ORGANIZATION_BLOCK OB 1
BEGIN
	// Check pointer immediates
	L		P#10.6
	__ASSERT==	__ACCU 1,	DW#16#00000056
	L		P#P 1.1
	__ASSERT==	__ACCU 1,	DW#16#80000009
	L		P#E 2.1
	__ASSERT==	__ACCU 1,	DW#16#81000011
	L		P#A 3.1
	__ASSERT==	__ACCU 1,	DW#16#82000019
	L		P#M 4.1
	__ASSERT==	__ACCU 1,	DW#16#83000021
	L		P#L 5.1
	__ASSERT==	__ACCU 1,	DW#16#86000029


	// Test address register instructions
	L		P#885.3
	LAR1
	L		P#886.2
	LAR2
	__ASSERT==	__ACCU 1,	P#886.2
	__ASSERT==	__ACCU 2,	P#885.3
	__ASSERT==	__AR 1,		P#885.3
	__ASSERT==	__AR 2,		P#886.2
	+AR1		P#1.1
	__ASSERT==	__AR 1,		P#886.4
	+AR2		P#5.1
	__ASSERT==	__AR 2,		P#891.3
	LAR1		P#12.3
	LAR2		P#32.1
	__ASSERT==	__AR 1,		P#12.3
	__ASSERT==	__AR 2,		P#32.1
	L		111
	L		222
	TAR1
	__ASSERT==	__ACCU 1,	P#12.3
	__ASSERT==	__ACCU 2,	222
	TAR2
	__ASSERT==	__ACCU 1,	P#32.1
	__ASSERT==	__ACCU 2,	P#12.3
	TAR1		LD 0
	TAR2		LD 4
	__ASSERT==	LD 0,		P#12.3
	__ASSERT==	LD 4,		P#32.1


	// Test indirect read
	L		0
	T		MD 100
	T		MD 104
	SET
	=		M 100.0
	=		M 100.2
	LAR1		P#100.0
	LAR2		P#104.0
	U		M [AR1, P#0.0]
	__ASSERT==	__STW VKE,	1
	U		M [AR1, P#0.1]
	__ASSERT==	__STW VKE,	0
	U		M [AR1, P#0.2]
	__ASSERT==	__STW VKE,	1
	U		M [AR1, P#0.3]
	__ASSERT==	__STW VKE,	0
	U		M [AR1, P#1.0]
	__ASSERT==	__STW VKE,	0
	U		M [AR2, P#0.0]
	__ASSERT==	__STW VKE,	0
	LAR1		P#100.1
	U		M [AR1, P#0.0]
	__ASSERT==	__STW VKE,	0
	U		M [AR1, P#0.1]
	__ASSERT==	__STW VKE,	1
	L		P#100.0
	T		LD 0
	U		M [LD 0]
	__ASSERT==	__STW VKE,	1
	L		P#100.1
	T		LD 0
	U		M [LD 0]
	__ASSERT==	__STW VKE,	0
	L		P#100.0
	T		LD 0
	L		MD [LD 0]
	__ASSERT==	__ACCU 1,	DW#16#05000000
	LAR1		P#M 100.0
	U		[AR1, P#0.0]
	__ASSERT==	__STW VKE,	1
	U		[AR1, P#0.1]
	__ASSERT==	__STW VKE,	0
	U		[AR1, P#0.2]
	__ASSERT==	__STW VKE,	1
	U		[AR1, P#0.3]
	__ASSERT==	__STW VKE,	0
	LAR1		P#M 100.0
	L		B [AR1, P#0.0]
	__ASSERT==	__ACCU 1,	DW#16#00000005
	L		W [AR1, P#0.0]
	__ASSERT==	__ACCU 1,	DW#16#00000500
	L		D [AR1, P#0.0]
	__ASSERT==	__ACCU 1,	DW#16#05000000


	// Test indirect write
	L		0
	T		MD 100
	T		MD 104
	SET
	=		M 100.0
	=		M 100.2
	LAR1		P#M 100.4
	=		[AR1, P#0.0]
	=		[AR1, P#0.1]
	L		MD 100
	__ASSERT==	__ACCU 1,	DW#16#35000000
	LAR1		P#M 100.0
	L		DW#16#ABCDEF12
	T		D [AR1, P#0.0]
	L		MD 100
	__ASSERT==	__ACCU 1,	DW#16#ABCDEF12
	T		D [AR1, P#1.0]
	L		MD 100
	__ASSERT==	__ACCU 1,	DW#16#ABABCDEF
	L		P#100.0
	T		LD 0
	L		DW#16#98765432
	T		MD [LD 0]
	L		MD 100
	__ASSERT==	__ACCU 1,	DW#16#98765432
	LAR1		P#100.0
	L		DW#16#12345678
	T		MD [AR1, P#0.0]
	L		MD 100
	__ASSERT==	__ACCU 1,	DW#16#12345678


	// Indirect counter access
	L		10
	T		LW 0
	L		Z [LW 0]
	__ASSERT==	__ACCU 1,	0
	SET
	ZV		Z 10
	CLR
	ZV		Z [LW 0]
	L		Z [LW 0]
	__ASSERT==	__ACCU 1,	1


	// Indirect timer access
	L		10
	T		LW 0
	L		T [LW 0]
	__ASSERT==	__ACCU 1,	0
	SET
	L		W#16#0999
	SI		T 10
	__SLEEP		50
	L		T [LW 0]
	__ASSERT<>	__ACCU 1,	0
	CLR
	L		W#16#0999
	SI		T [LW 0]
	L		T [LW 0]
	__SLEEP		50
	L		T [LW 0]
	__ASSERT==	__ACCU 1,	__ACCU 2


	CALL FB 1, DB 1 (
		IN_VAL_0	:= 6666,
		IN_VAL_1	:= 6767,
		ZERO_PTR_VAL	:= DW#16#0,
		ONE_PTR_VAL	:= DW#16#8,
	)

	CALL FC 1 (
		IN_VAL_0	:= 5555,
		IN_VAL_1	:= 5656,
	)

	CALL FC 2


	CALL SFC 46 // STOP CPU
END_ORGANIZATION_BLOCK


FUNCTION_BLOCK FB 1
	VAR_INPUT
		IN_VAL_0	: INT;
		IN_VAL_1	: INT;
		ZERO_PTR_VAL	: DWORD;
		ONE_PTR_VAL	: DWORD;
	END_VAR
BEGIN
	L		P##IN_VAL_0
	__ASSERT==	__ACCU 1,	DW#16#85000000
	L		P##IN_VAL_1
	__ASSERT==	__ACCU 1,	DW#16#85000010


	L		DW#16#11223344
	T		MD 0
	L		DW#16#55667788
	T		MD 4
	L		MD [#ZERO_PTR_VAL]
	__ASSERT==	__ACCU 1,	DW#16#11223344
	L		MD [#ONE_PTR_VAL]
	__ASSERT==	__ACCU 1,	DW#16#22334455


	L		DW#16#AABBCCDD
	T		MD 1
	L		1
	T		MW 12
	L		2
	T		MW 14
	CALL FB 2, DB 2 (
		IN_VAL_0	:= MD [#ONE_PTR_VAL],
		DB_VAL		:= DB [MW 14],
		FC_VAL		:= FC [MW 12],
		FB_VAL		:= FB [MW 12],
	)


	// Test all memory-indirect accesses
	AUF		DB 1
	L		P#8.0
	T		LD 0
	U		E [LD 0]
	=		E [LD 0]
	U		A [LD 0]
	=		A [LD 0]
	U		L [LD 0]
	=		L [LD 0]
	U		DIX [LD 0]
	=		DIX [LD 0]
	U		DBX [LD 0]
	=		DBX [LD 0]
	L		EB [LD 0]
	T		EB [LD 0]
	L		AB [LD 0]
	T		AB [LD 0]
	L		MB [LD 0]
	T		MB [LD 0]
	L		LB [LD 0]
	T		LB [LD 0]
	L		PEB [LD 0]
	T		PAB [LD 0]
	L		DBB [LD 0]
	T		DBB [LD 0]
	L		DIB [LD 0]
	T		DIB [LD 0]
	L		EW [LD 0]
	T		EW [LD 0]
	L		AW [LD 0]
	T		AW [LD 0]
	L		MW [LD 0]
	T		MW [LD 0]
	L		LW [LD 0]
	T		LW [LD 0]
	L		PEW [LD 0]
	T		PAW [LD 0]
	L		DBW [LD 0]
	T		DBW [LD 0]
	L		DIW [LD 0]
	T		DIW [LD 0]
	L		ED [LD 0]
	T		ED [LD 0]
	L		AD [LD 0]
	T		AD [LD 0]
	L		MD [LD 0]
	T		MD [LD 0]
	L		LD [LD 0]
	T		LD [LD 0]
	L		PED [LD 0]
	T		PAD [LD 0]
	L		DBD [LD 0]
	T		DBD [LD 0]
	L		DID [LD 0]
	T		DID [LD 0]
	L		0
	T		LW 0
	L		T [LW 0]
	L		Z [LW 0]

	// Test all register-indirect accesses
	AUF		DB 1
	LAR1		P#8.0
	U		E [AR1, P#0.0]
	=		E [AR1, P#0.0]
	LAR1		P#E 8.0
	U		[AR1, P#0.0]
	=		[AR1, P#0.0]
	LAR1		P#8.0
	U		A [AR1, P#0.0]
	=		A [AR1, P#0.0]
	LAR1		P#A 8.0
	U		[AR1, P#0.0]
	=		[AR1, P#0.0]
	LAR1		P#8.0
	U		M [AR1, P#0.0]
	=		M [AR1, P#0.0]
	LAR1		P#M 8.0
	U		[AR1, P#0.0]
	=		[AR1, P#0.0]
	LAR1		P#8.0
	U		L [AR1, P#0.0]
	=		L [AR1, P#0.0]
	LAR1		P#L 8.0
	U		[AR1, P#0.0]
	=		[AR1, P#0.0]
	LAR1		P#8.0
	U		DIX [AR1, P#0.0]
	=		DIX [AR1, P#0.0]
	LAR1		P#DIX 8.0
	U		[AR1, P#0.0]
	=		[AR1, P#0.0]
	LAR1		P#8.0
	U		DBX [AR1, P#0.0]
	=		DBX [AR1, P#0.0]
	LAR1		P#DBX 8.0
	U		[AR1, P#0.0]
	=		[AR1, P#0.0]

	LAR1		P#8.0
	L		EB [AR1, P#0.0]
	T		EB [AR1, P#0.0]
	LAR1		P#E 8.0
	L		B [AR1, P#0.0]
	T		B [AR1, P#0.0]
	LAR1		P#8.0
	L		AB [AR1, P#0.0]
	T		AB [AR1, P#0.0]
	LAR1		P#A 8.0
	L		B [AR1, P#0.0]
	T		B [AR1, P#0.0]
	LAR1		P#8.0
	L		MB [AR1, P#0.0]
	T		MB [AR1, P#0.0]
	LAR1		P#M 8.0
	L		B [AR1, P#0.0]
	T		B [AR1, P#0.0]
	LAR1		P#8.0
	L		LB [AR1, P#0.0]
	T		LB [AR1, P#0.0]
	LAR1		P#L 8.0
	L		B [AR1, P#0.0]
	T		B [AR1, P#0.0]
	LAR1		P#8.0
	L		PEB [AR1, P#0.0]
	T		PAB [AR1, P#0.0]
	LAR1		P#P 8.0
	L		B [AR1, P#0.0]
	T		B [AR1, P#0.0]
	LAR1		P#8.0
	L		DBB [AR1, P#0.0]
	T		DBB [AR1, P#0.0]
	LAR1		P#DBX 8.0
	L		B [AR1, P#0.0]
	T		B [AR1, P#0.0]
	LAR1		P#8.0
	L		DIB [AR1, P#0.0]
	T		DIB [AR1, P#0.0]
	LAR1		P#DIX 8.0
	L		B [AR1, P#0.0]
	T		B [AR1, P#0.0]

	LAR1		P#8.0
	L		EW [AR1, P#0.0]
	T		EW [AR1, P#0.0]
	LAR1		P#E 8.0
	L		W [AR1, P#0.0]
	T		W [AR1, P#0.0]
	LAR1		P#8.0
	L		AW [AR1, P#0.0]
	T		AW [AR1, P#0.0]
	LAR1		P#A 8.0
	L		W [AR1, P#0.0]
	T		W [AR1, P#0.0]
	LAR1		P#8.0
	L		MW [AR1, P#0.0]
	T		MW [AR1, P#0.0]
	LAR1		P#M 8.0
	L		W [AR1, P#0.0]
	T		W [AR1, P#0.0]
	LAR1		P#8.0
	L		LW [AR1, P#0.0]
	T		LW [AR1, P#0.0]
	LAR1		P#L 8.0
	L		W [AR1, P#0.0]
	T		W [AR1, P#0.0]
	LAR1		P#8.0
	L		PEW [AR1, P#0.0]
	T		PAW [AR1, P#0.0]
	LAR1		P#P 8.0
	L		W [AR1, P#0.0]
	T		W [AR1, P#0.0]
	LAR1		P#8.0
	L		DBW [AR1, P#0.0]
	T		DBW [AR1, P#0.0]
	LAR1		P#DBX 8.0
	L		W [AR1, P#0.0]
	T		W [AR1, P#0.0]
	LAR1		P#8.0
	L		DIW [AR1, P#0.0]
	T		DIW [AR1, P#0.0]
	LAR1		P#DIX 8.0
	L		W [AR1, P#0.0]
	T		W [AR1, P#0.0]

	LAR1		P#8.0
	L		ED [AR1, P#0.0]
	T		ED [AR1, P#0.0]
	LAR1		P#E 8.0
	L		D [AR1, P#0.0]
	T		D [AR1, P#0.0]
	LAR1		P#8.0
	L		AD [AR1, P#0.0]
	T		AD [AR1, P#0.0]
	LAR1		P#A 8.0
	L		D [AR1, P#0.0]
	T		D [AR1, P#0.0]
	LAR1		P#8.0
	L		MD [AR1, P#0.0]
	T		MD [AR1, P#0.0]
	LAR1		P#M 8.0
	L		D [AR1, P#0.0]
	T		D [AR1, P#0.0]
	LAR1		P#8.0
	L		LD [AR1, P#0.0]
	T		LD [AR1, P#0.0]
	LAR1		P#L 8.0
	L		D [AR1, P#0.0]
	T		D [AR1, P#0.0]
	LAR1		P#8.0
	L		PED [AR1, P#0.0]
	T		PAD [AR1, P#0.0]
	LAR1		P#P 8.0
	L		D [AR1, P#0.0]
	T		D [AR1, P#0.0]
	LAR1		P#8.0
	L		DBD [AR1, P#0.0]
	T		DBD [AR1, P#0.0]
	LAR1		P#DBX 8.0
	L		D [AR1, P#0.0]
	T		D [AR1, P#0.0]
	LAR1		P#8.0
	L		DID [AR1, P#0.0]
	T		DID [AR1, P#0.0]
	LAR1		P#DIX 8.0
	L		D [AR1, P#0.0]
	T		D [AR1, P#0.0]
END_FUNCTION_BLOCK


FUNCTION_BLOCK FB 2
	VAR_INPUT
		IN_VAL_0	: DWORD;
		DB_VAL		: BLOCK_DB;
		FC_VAL		: BLOCK_FC;
		FB_VAL		: BLOCK_FB;
	END_VAR
BEGIN
	L		#IN_VAL_0
	__ASSERT==	__ACCU 1,	DW#16#AABBCCDD

	AUF		#DB_VAL
	L		DBD 0
	L		#IN_VAL_0
	__ASSERT==	__ACCU 1,	__ACCU 2
END_FUNCTION_BLOCK


FUNCTION FC 1 : VOID
	VAR_INPUT
		IN_VAL_0	: INT;
		IN_VAL_1	: INT;
	END_VAR
BEGIN
	L		P##IN_VAL_0
	UD		DW#16#FFF80000
	__ASSERT==	__ACCU 1,	DW#16#87000000
	L		P##IN_VAL_1
	UD		DW#16#FFF80000
	__ASSERT==	__ACCU 1,	DW#16#87000000
END_FUNCTION


FUNCTION FC 2 : VOID
TITLE =Extended address register instruction tests
BEGIN
	// Open the data blocks
	AUF		DB 3
	AUF		DI 3
	// Initialize the memory areas
	L		P#42.0
	T		MD 0
	L		P#43.0
	T		LD 0
	L		P#44.0
	T		DBD 0
	L		P#45.0
	T		DID 4
	LAR2		P#46.0
	L		P#47.0
	T		MD 42


	// Test LAR1
	LAR1		MD 0
	__ASSERT==	__AR 1,		P#42.0
	LAR1		LD 0
	__ASSERT==	__AR 1,		P#43.0
	LAR1		DBD 0
	__ASSERT==	__AR 1,		P#44.0
	LAR1		DID 4
	__ASSERT==	__AR 1,		P#45.0
	LAR1		AR2
	__ASSERT==	__AR 1,		P#46.0

	// Test LAR2
	LAR2		MD 0
	__ASSERT==	__AR 2,		P#42.0
	LAR2		LD 0
	__ASSERT==	__AR 2,		P#43.0
	LAR2		DBD 0
	__ASSERT==	__AR 2,		P#44.0
	LAR2		DID 4
	__ASSERT==	__AR 2,		P#45.0

	// Test TAR1
	LAR1		P#142.7
	LAR2		P#143.1
	TAR1		MD 0
	__ASSERT==	MD 0,		P#142.7
	TAR1		LD 0
	__ASSERT==	LD 0,		P#142.7
	TAR1		DBD 0
	__ASSERT==	DBD 0,		P#142.7
	TAR1		DID 4
	__ASSERT==	DID 4,		P#142.7
	TAR1		AR2
	__ASSERT==	__AR 2,		P#142.7

	// Test TAR2
	LAR1		P#142.7
	LAR2		P#143.1
	TAR2		MD 0
	__ASSERT==	MD 0,		P#143.1
	TAR2		LD 0
	__ASSERT==	LD 0,		P#143.1
	TAR2		DBD 0
	__ASSERT==	DBD 0,		P#143.1
	TAR2		DID 4
	__ASSERT==	DID 4,		P#143.1


	// Test offset wrapping
	LAR1		P#41.7
	L		MD [AR1,P#0.1]
	__ASSERT==	__ACCU 1,	P#47.0
END_FUNCTION


DATA_BLOCK DB 1
	FB 1
BEGIN
	IN_VAL_0	:= 88;
	IN_VAL_1	:= 99;
END_DATA_BLOCK


DATA_BLOCK DB 2
	FB 2
BEGIN
END_DATA_BLOCK


DATA_BLOCK DB 3
STRUCT
	pointer_0 : DWORD;
	pointer_1 : DWORD;
END_STRUCT;
BEGIN
	pointer_0 := DW#16#0;
	pointer_1 := DW#16#0;
END_DATA_BLOCK
